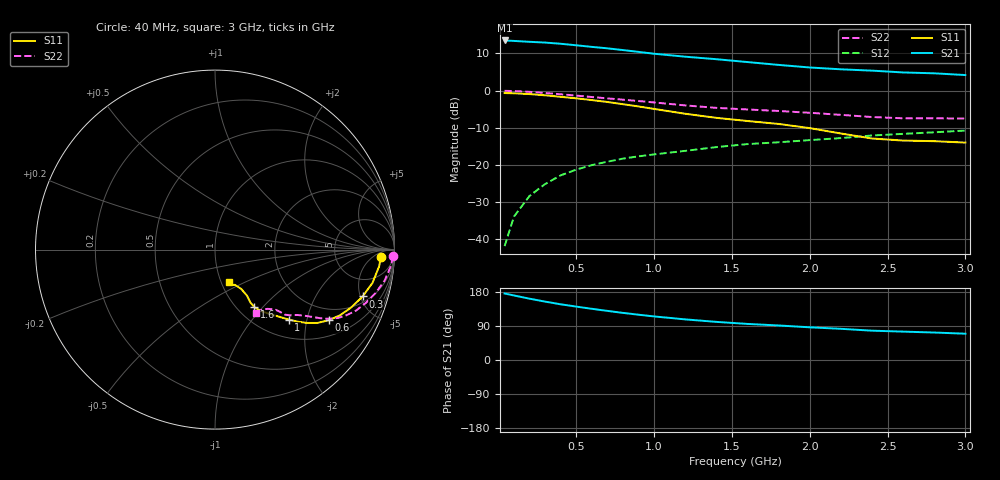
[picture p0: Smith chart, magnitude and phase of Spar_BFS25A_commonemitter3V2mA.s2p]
! Filename:  BFS25AJ.S2P  Version:  4.0
! NXP part #: BFS25A  Date: Jun 1994
! Bias condition: Vce=3V, Ic=2mA
#  MHz  S  MA  R  50
! Freq  S11  S21  S12  S22  !GUM [dB]
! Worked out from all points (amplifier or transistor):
!   21 points, 40 MHz to 3 GHz, reference 50 ohm
!   highest |S21| = 13.5 dB at 40 MHz (marker M1)
!   |S21| within 3 dB of that: start of sweep to 883.9 MHz
!   unconditionally stable (mu >= 1): 1.811 GHz to end of sweep
!   at 300 MHz: K = 0.30, MSG = 19.1 dB, |S12| = -25.2 dB
!   at 1 GHz: K = 0.73, MSG = 13.6 dB, |S12| = -17.2 dB
!   at 3 GHz: K = 1.11, MAG = 5.5 dB, |S12| = -10.8 dB
!   lowest NFmin = 2.50 dB at 500 MHz
!   S11 on the Smith chart (normalised r, x): 40 MHz: 20, -11; 300 MHz: 2.56, -5.24; 600 MHz: 1.53, -2.71; 1 GHz: 1.36, -1.56; 1.6 GHz: 1.19, -0.90; 3 GHz: 1.09, -0.41
40  0.926 -2.5  4.735 175.5  0.008 88.2  0.992 -2.1
100  0.919 -5.9  4.667 170.3  0.02 83.9  0.985 -5.2
200  0.897 -11.9  4.541 161.8  0.038 79.7  0.961 -10.3
300  0.863 -17.6  4.434 154.1  0.055 75.8  0.927 -15.1
400  0.824 -23.1  4.274 147.0  0.072 72.8  0.892 -19.4
500  0.786 -27.8  4.077 140.9  0.086 70.1  0.856 -23.4
600  0.745 -31.9  3.881 135.1  0.099 67.9  0.819 -26.5
700  0.702 -35.6  3.708 129.6  0.11 66.5  0.785 -29.0
800  0.655 -38.6  3.514 124.3  0.121 65.3  0.754 -30.7
900  0.611 -41.1  3.322 119.5  0.13 63.8  0.723 -32.2
1000  0.566 -43.5  3.136 115.0  0.138 62.6  0.692 -33.4
1200  0.487 -48.4  2.861 107.2  0.154 60.6  0.631 -35.9
1400  0.429 -53.1  2.647 100.6  0.173 59.3  0.585 -38.5
1600  0.389 -55.6  2.421 95.2  0.19 58.2  0.556 -41.2
1800  0.355 -56.2  2.217 91.1  0.201 58.1  0.531 -43.0
2000  0.312 -55.2  2.047 86.3  0.215 57.4  0.502 -43.7
2200  0.264 -56.3  1.935 82.3  0.229 56.9  0.471 -45.0
2400  0.226 -60.4  1.856 77.4  0.248 55.7  0.44 -48.6
2600  0.212 -67.6  1.755 74.9  0.261 54.6  0.423 -53.0
2800  0.208 -70.3  1.708 72.5  0.274 55.1  0.423 -55.8
3000  0.199 -67.0  1.618 69.4  0.289 54.5  0.42 -57.0
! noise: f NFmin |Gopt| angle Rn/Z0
500  2.5  0.775  4  2.2
1000  2.5  0.731  10  2.2
2000  3  0.662  27  1.6
